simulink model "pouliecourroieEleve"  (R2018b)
settings: Solver=VariableStepAuto  StartTime=0.0  StopTime=10.0  RelTol=1e-3
libraries: simulink x1

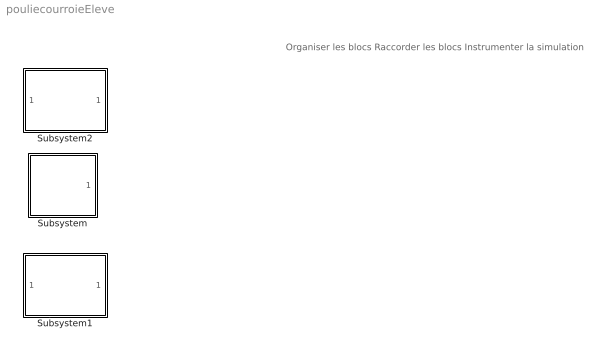
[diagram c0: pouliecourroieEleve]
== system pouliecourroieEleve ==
  note: Organiser les blocs Raccorder les blocs Instrumenter la simulation
  Subsystem : Subsystem  mask{acc=0, wm=0}
      mask prompts: acc "Accélération (rad.s-2)"; wm "Vitesse angulaire (rad.s-1)"
  Subsystem1 : Subsystem  mask{R=0}
      mask prompts: R "Rayon (m)"
  Subsystem2 : Subsystem  mask{R=0}
      mask prompts: R "Rayon (m)"

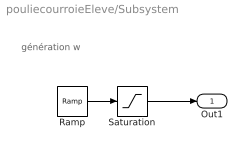
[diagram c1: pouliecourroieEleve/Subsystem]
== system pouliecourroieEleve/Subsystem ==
  note: génération w
  Ramp : simulink/Sources/Ramp  slope=acc  start=0  InitialOutput=0
  Saturation : Saturate  UpperLimit=wm
  Out1 : Outport
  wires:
  Ramp/1 -> Saturation/1
  Saturation/1 -> Out1/1

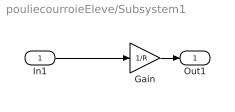
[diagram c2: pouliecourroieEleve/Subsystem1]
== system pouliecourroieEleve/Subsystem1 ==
  In1 : Inport
  Gain : Gain  Gain=1/R
  Out1 : Outport
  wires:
  Gain/1 -> Out1/1
  In1/1 -> Gain/1

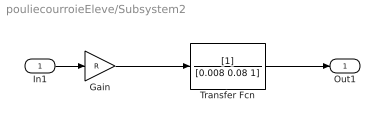
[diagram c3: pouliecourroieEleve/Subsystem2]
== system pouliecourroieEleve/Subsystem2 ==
  In1 : Inport
  Gain : Gain  Gain=R
  Transfer Fcn : TransferFcn  Denominator=[0.008 0.08 1]
  Out1 : Outport
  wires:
  In1/1 -> Gain/1
  Gain/1 -> Transfer Fcn/1
  Transfer Fcn/1 -> Out1/1
